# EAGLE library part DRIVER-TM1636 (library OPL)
The led Special drive control circuit
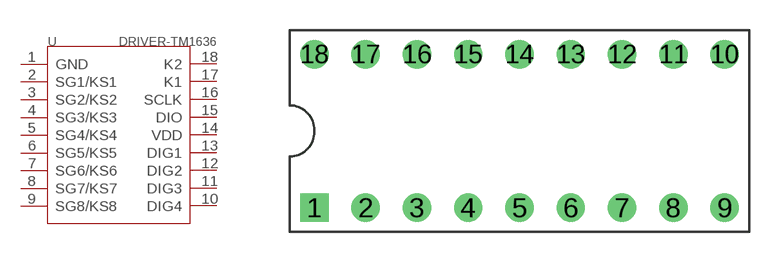
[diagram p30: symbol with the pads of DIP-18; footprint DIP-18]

Designator prefix U

## DRIVER-TM1636-310040002  [DIP-18]
1  GND
2  SG1/KS1
3  SG2/KS2
4  SG3/KS3
5  SG4/KS4
6  SG5/KS5
7  SG6/KS6
8  SG7/KS7
9  SG8/KS8
10  DIG4
11  DIG3
12  DIG2
13  DIG1
14  VDD
15  DIO
16  SCLK
17  K1
18  K2

## Footprint DIP-18 (pad centres in mm)
drill 0.9 pad 1.4 square: 1 -10.16,-3.81
drill 0.9 pad 1.4: 2 -7.62,-3.81; 3 -5.08,-3.81; 4 -2.54,-3.81; 5 0,-3.81; 6 2.54,-3.81; 7 5.08,-3.81; 8 7.62,-3.81; 9 10.16,-3.81; 10 10.16,3.81; 11 7.62,3.81; 12 5.08,3.81; 13 2.54,3.81; 14 0,3.81; 15 -2.54,3.81; 16 -5.08,3.81; 17 -7.62,3.81; 18 -10.16,3.81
